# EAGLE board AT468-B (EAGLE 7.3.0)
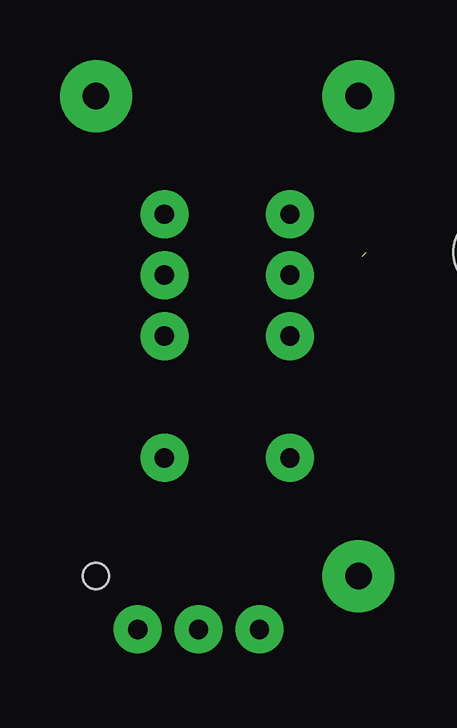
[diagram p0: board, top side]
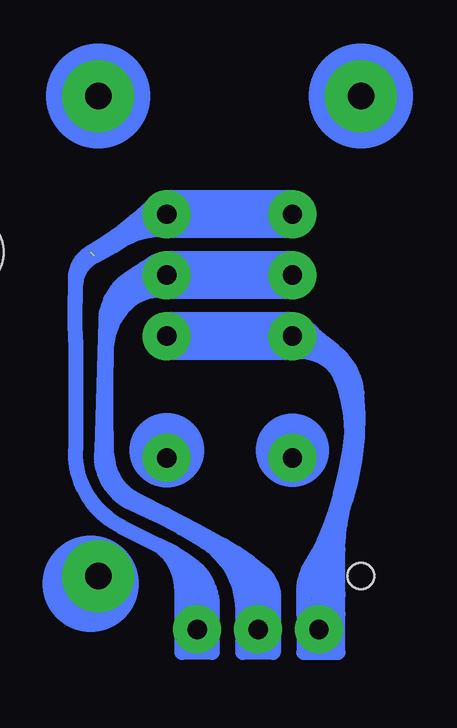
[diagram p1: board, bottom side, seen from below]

No outline drawn. Coordinates in mm, seen from the top.
Copper layers (1*16): Top 0.035mm / dielectric 1.5mm / Bottom 0.035mm
Design rules "default": minimum track width 10mil, minimum drill 24mil, track to track 8mil, track to pad 8mil, pad to pad 8mil, via to via 8mil, smd to smd 8mil, copper to edge 40mil, drill to drill 8mil, minimum pad ring 10mil, minimum via ring 8mil, stop-mask expansion 4mil, vias tented up to drill 0mil, thermal gap 10mil
Holes 3.2 mm at 19.05,17.14
Holes 1.1 mm at 2.54,3.65

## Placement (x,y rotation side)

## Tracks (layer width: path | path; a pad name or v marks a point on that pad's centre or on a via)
S$1
  Bottom 0.635: 5.24,13.02 5.08,13.02 | 5.08,13.02 4.76,13.02 | 5.24,13.02 arc1 4.45,13.02 arc53 3.81,12.7 | 5.4,13.02 5.24,13.02 | 5.08,13.02 arc65 3.33,11.91
S$2
  Bottom 0.635: 3.65,5.08 4.45,3.17
S$3  (via drill 0.8 pad 2)
  other vias: 10.64,8.57
S$4  (via drill 1.1 pad 3)
  other vias: 13.49,3.65
S$5  (via drill 1.1 pad 3)
  other vias: 2.54,23.65
S$6  (via drill 1.1 pad 3)
  other vias: 13.49,23.65
S$7
  Bottom 0.635: 3.49,2.06 arc-28 4.13,2.7 4.92,2.06 | 4.92,2.06 4.92,0.48 3.49,0.48 3.49,2.86 | 4.92,2.06 4.92,2.86 | 4.92,2.86 arc180 3.49,2.86 | 3.49,2.86 3.49,4.76 arc17 3.17,6.83 arc-23 2.7,11.27 arc-47 3.65,13.02 arc6 4.92,14.13 | 4.92,2.86 4.92,3.02 arc32 4.6,4.13 arc-14 3.65,6.19 arc-7 3.02,8.73 arc-36 3.49,12.22 4.13,13.18
S$8  (via drill 0.8 pad 2)
  Bottom 2: v5.4,16.19 v10.64,16.19
S$9  (via drill 0.8 pad 2)
  Bottom 2: v5.4,18.73 v10.64,18.73
S$10
  Bottom 0.635: 3.81,3.17 3.81,4.45
S$11
  Bottom 0.635: 3.81,3.02 4.45,3.02
S$12
  Bottom 0.635: 10.32,15.56 10.95,15.56 arc-41 12.22,15.08 arc-48 13.18,13.02 arc-1 13.18,9.05 arc-18 13.02,8.1 arc-46 11.91,6.83 arc3 8.26,4.92 arc12 6.67,3.81 arc57 6.19,2.54
S$13
  Bottom 0.635: 6.19,2.7 6.19,0.48 7.46,0.48 7.46,2.22 arc-58 9.05,5.08 arc-8 12.06,6.67 arc73 13.34,8.89 13.18,14.29 arc54 12.22,16.03 arc2 11.27,16.67 arc43 10.48,16.83
S$14
  Bottom 0.635: 12.54,15.24 11.43,16.03
S$15
  Bottom 0.635: 6.67,0.95 6.67,3.17
S$16
  Bottom 0.635: 7.94,4.6 6.83,3.33
S$17
  Bottom 0.635: 7.14,3.81 6.99,0.79
S$18  (1 unrouted)
  Bottom 0.635: 10.79,18.1 arc-33 12.54,17.62 arc4 13.65,16.99 arc-61 14.45,15.72 arc-3 14.45,13.49 14.45,8.89 arc-65 12.54,5.71 10.95,4.92 | 11.27,19.05 arc13 13.81,17.14 arc-59 14.45,16.03 14.45,15.08 | 10.95,4.92 10.32,4.6 arc-8 9.84,4.29 arc61 8.73,2.38 8.73,0.48 10,0.48 10,3.02 arc-53 10.95,4.92
S$19  (via drill 0.8 pad 2)
  Bottom 2: v5.4,13.65 v10.64,13.65
S$20
  Bottom 0.635: 10.95,18.73 12.7,17.62
S$22
  Bottom 0.635: 9.21,0.79 9.21,3.17
S$23
  Bottom 0.635: 9.84,3.97 9.53,3.33 9.53,0.95
S$24  (via drill 0.8 pad 2)
  other vias: 5.4,8.57
S$359  (via drill 0.8 pad 2)
  other vias: 4.29,1.43
S$360  (via drill 0.8 pad 2)
  other vias: 6.83,1.43
S$361  (via drill 0.8 pad 2)
  other vias: 9.37,1.43
(copper drawn outside any net)
  shapes: Bottom area x1, Bottom circle x5

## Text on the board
tValues: O2 | JLCJLCJLCJLC | AT468B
